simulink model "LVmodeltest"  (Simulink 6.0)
settings: Solver=ode45  StartTime=0.0  StopTime=10.0  RelTol=1e-3

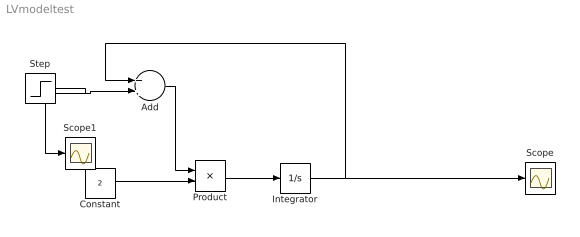
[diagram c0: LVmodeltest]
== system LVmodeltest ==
  Add : Sum  OutScaling=2^-10
  Constant : Constant  Value=2
  Integrator : Integrator
  Product : Product
  Scope : Scope
  Scope1 : Scope
  Step : Step  Time=8  Before=1  After=0  SampleTime=0
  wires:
  Integrator/1 -> Scope/1, Add/1
  Constant/1 -> Product/2
  Product/1 -> Integrator/1
  Step/1 -> Add/2, Scope1/1
  Add/1 -> Product/1
